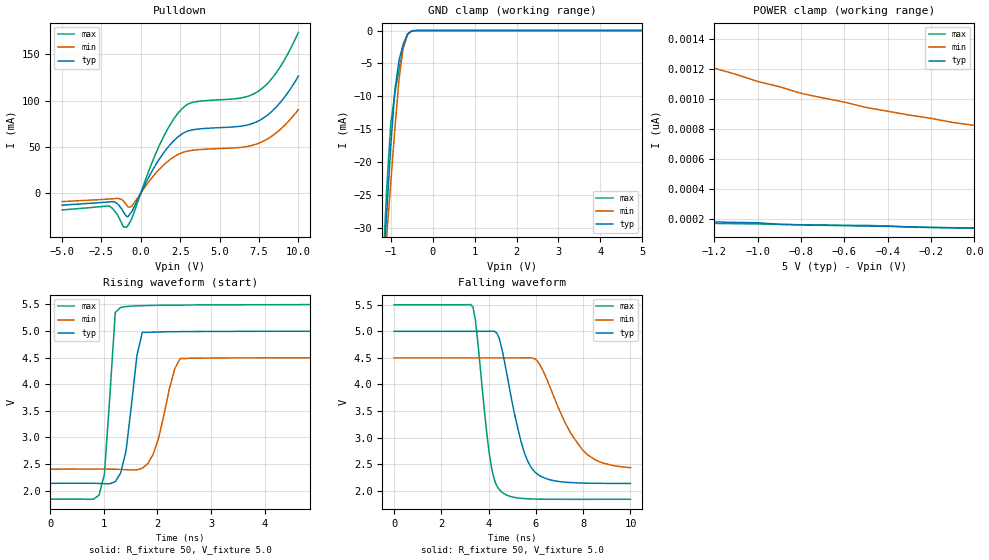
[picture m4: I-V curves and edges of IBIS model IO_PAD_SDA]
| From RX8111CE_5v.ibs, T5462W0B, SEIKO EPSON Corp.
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[Model]   IO_PAD_SDA
Model_type I/O_open_drain
Enable Active-High
Polarity Non-Inverting
Vinh=4.4
Vinl=0.9
Vmeas=2.5
Vref=5.5
Rref=5000
C_comp   2.5p   2.0p   3.0p
[Temperature Range] 25   105   -40
[Voltage Range]   5.0   4.5   5.5
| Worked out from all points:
|   slope of the pulldown table from 0 to 0.75 V, typ, clamps not added: 30.2 ohm
|   GND clamp passes 1 mA (typ) near -0.63 V on its own axis
|   falling waveform, R_fixture 50, V_fixture 5.0: 20-80 % time 848ps typ, 1.37ns min, 525ps max; typ from 5 V to 2.14 V
|   rising waveform, R_fixture 50, V_fixture 5.0: 20-80 % time 200ps typ, 300ps min, 147ps max; typ from 2.14 V to 5 V
[Pulldown]
-5V       -13.16mA   -9.279mA   -18.37mA
-2V       -9.66mA    -6.523mA   -13.96mA
-1.5V     -11.48mA   -5.863mA   -23.2mA
-1.1V     -20.65mA   -8.791mA   -36.89mA
-900mV    -25.65mA   -13.16mA   -36.96mA
-600mV    -20.79mA   -14.82mA   -28.65mA
1.1V      34.77mA    24.37mA    48.65mA
2.4V      61.28mA    41.98mA    87.2mA
3.3V      68.39mA    46.26mA    98.05mA
7.4V      77.39mA    53.3mA     109.5mA
8.6V      93.1mA     65.14mA    130.2mA
10V       126.3mA    90.2mA     173.8mA
[GND Clamp]
-5V       -462.3mA   -375.8mA   -568.7mA
-1.2V     -38.9mA    -40.16mA   -37.89mA
-1.1V     -28.19mA   -31.69mA   -24.51mA
-1V       -17.59mA   -23.23mA   -14.19mA
-900mV    -8.973mA   -14.82mA   -9.505mA
-800mV    -4.446mA   -7.292mA   -5.814mA
-700mV    -2.032mA   -2.408mA   -2.637mA
-600mV    -545.2uA   -567.5uA   -605.7uA
-500mV    -56.87uA   -91.02uA   -35.51uA
5V        140.1pA    943.1pA    125.5pA
[POWER Clamp]
-5V       376.5pA    7.023nA    8.229uA
-4.7V     356.5pA    6.142nA    4.18nA
-4.6V     351.1pA    5.863nA    287.4pA
-4.5V     342pA      5.597nA    241.9pA
-3.9V     305.6pA    4.217nA    227.4pA
-3.7V     277.4pA    3.817nA    222.8pA
-1.7V     198.3pA    1.477nA    182.8pA
-1.6V     192.8pA    1.412nA    181pA
-1.2V     180.1pA    1.204nA    170.1pA
-800mV    160.1pA    1.037nA    161pA
-500mV    152.8pA    943.1pA    156.4pA
0V        140.1pA    823.5pA    138.2pA
[Falling Waveform]
R_fixture=50
V_fixture=5.0
V_fixture_min=4.5
V_fixture_max=5.5
0s        5V         4.5V       5.5V
3.333ns   5V         4.5V       5.458V
3.434ns   5V         4.5V       5.225V
4.04ns    5.002V     4.5V       2.65V
4.242ns   5.001V     4.5V       2.2V
4.545ns   4.696V     4.5V       1.977V
5.354ns   2.954V     4.501V     1.858V
5.96ns    2.35V      4.482V     1.843V
7.98ns    2.144V     2.764V     1.838V
10ns      2.136V     2.433V     1.838V
[Rising Waveform]
R_fixture=50
V_fixture=5.0
V_fixture_min=4.5
V_fixture_max=5.5
0s        2.136V     2.401V     1.837V
909.1ps   2.134V     2.403V     1.913V
1.01ns    2.129V     2.403V     2.309V
1.212ns   2.166V     2.401V     5.35V
1.313ns   2.33V      2.397V     5.446V
1.414ns   2.75V      2.392V     5.462V
1.717ns   4.978V     2.421V     5.478V
1.919ns   4.98V      2.683V     5.483V
2.424ns   4.99V      4.484V     5.489V
10ns      5V         4.5V       5.5V
[Ramp]
R_load=50
dV/dt_r   1.719E+0/1.880E-10   1.259E+0/2.912E-10   2.198E+0/1.390E-10
dV/dt_f   1.718E+0/8.435E-10   1.240E+0/1.371E-9   2.197E+0/5.213E-10
|[End   IO_PAD_SDA
